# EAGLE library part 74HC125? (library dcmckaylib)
Quad 3-State Buffer
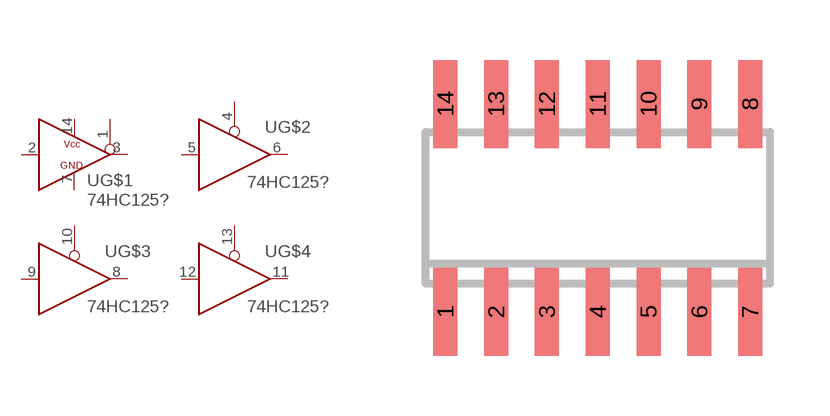
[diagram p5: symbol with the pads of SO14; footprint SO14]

Designator prefix U; gates G$1=BUFFERWINVERT2 G$2=BUFFERWINVERT G$3=BUFFERWINVERT G$4=BUFFERWINVERT

## 74HC125M  [SO14]
1  G$1:ENABLE  in
2  G$1:IN  in
3  G$1:OUT  out
4  G$2:ENABLE  in
5  G$2:IN  in
6  G$2:OUT  out
7  G$1:GND  pwr
8  G$3:OUT  out
9  G$3:IN  in
10  G$3:ENABLE  in
11  G$4:OUT  out
12  G$4:IN  in
13  G$4:ENABLE  in
14  G$1:VCC  pwr

## Footprint SO14 (pad centres in mm)
Small Outline Package 14
smd 0.6 x 2.2: 1 -3.81,-2.6; 2 -2.54,-2.6; 3 -1.27,-2.6; 4 0,-2.6; 5 1.27,-2.6; 6 2.54,-2.6; 7 3.81,-2.6; 8 3.81,2.6; 9 2.54,2.6; 10 1.27,2.6; 11 0,2.6; 12 -1.27,2.6; 13 -2.54,2.6; 14 -3.81,2.6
